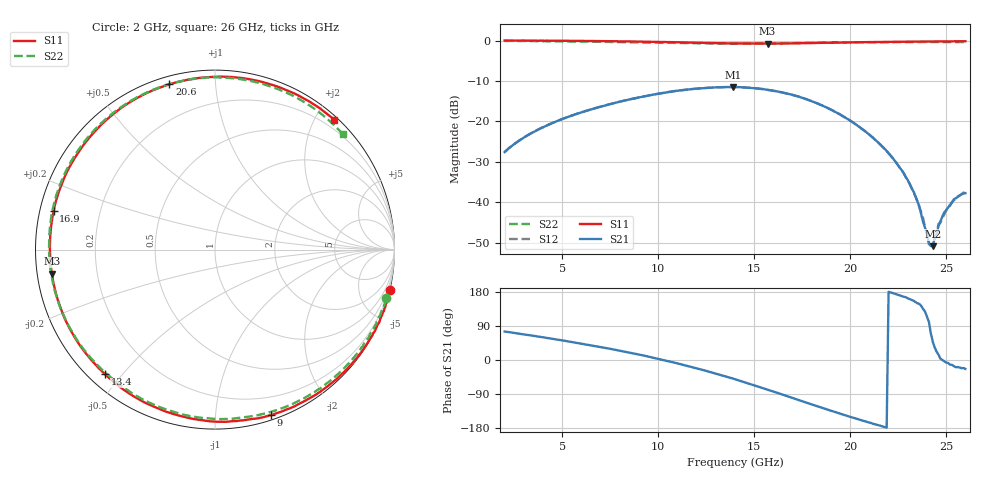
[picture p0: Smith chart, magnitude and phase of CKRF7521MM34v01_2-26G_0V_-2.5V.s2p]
! CHUO DENSHI KOGYO Co.,Ltd.
! 1. March 2016
! CKRF7521MM34
! N-channel HJ-FET
! Vds = 0 V Vgs = -2.5 V
# Hz S  MA  R 50
!  f  S11  S21  S12  S22
!  Hz  MAG  ANG  MAG  ANG  MAG  ANG  MAG  ANG
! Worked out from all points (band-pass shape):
!   241 points, 2 GHz to 26 GHz, reference 50 ohm
!   highest |S21| = -11.48 dB at 13.9 GHz (marker M1); lowest = -50.9 dB at 24.3 GHz (marker M2)
!   |S21| within 3 dB of the highest: 8.573 GHz to 17.71 GHz (9.138 GHz wide, 69.5 % of centre)
!   lowest |S11| = -0.7 dB at 15.7 GHz (marker M3), VSWR 23.56, Z = 2.13 - j3.69 ohm
!   |S11| at or under -10 dB: nowhere
!   |S22| runs from -0.7 to -0.1 dB; largest |S21 - S12| = 0.00066
!   S11 on the Smith chart (normalised r, x): 2 GHz: -0.06, -8.68; 9 GHz: 0.04, -1.39; 13.4 GHz: 0.05, -0.45; 16.9 GHz: 0.04, +0.12; 20.6 GHz: 0.04, +0.76; 26 GHz: 0.05, +2.28
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2e9  1.002 -13.1  0.04171 75.2  0.04194 75.2  0.9908 -15.9
3.8e9  0.999 -25.6  0.08043 61.5  0.08046 61.5  0.9834 -30.5
6e9  0.9913 -42.7  0.1294 43.3  0.1297 43.3  0.9724 -49.4
9e9  0.9729 -71.4  0.1985 14.4  0.1985 14.4  0.9497 -78.5
1e10  0.963 -82.9  0.2202 3.3  0.22 3.2  0.9433 -89.3
1.18e10  0.9432 -106.8  0.252 -19.3  0.2521 -19.3  0.929 -110.8
1.34e10  0.9262 -131.4  0.2655 -41.6  0.2658 -41.7  0.9181 -132.0
1.39e10  0.9228 -139.7  0.2667 -49.3  0.2667 -49.3  0.9186 -139.1
1.4e10  0.9231 -141.3  0.2661 -50.9  0.2662 -50.9  0.9181 -140.5
1.57e10  0.9186 -171.5  0.2461 -78.3  0.246 -78.2  0.9213 -166.5
1.69e10  0.9246 166.6  0.2162 -98.4  0.216 -98.3  0.9267 173.9
1.8e10  0.9334 146.9  0.1779 -117.3  0.1779 -117.2  0.9368 155.5
1.93e10  0.9455 125.0  0.1282 -138.7  0.1281 -138.8  0.9467 133.7
2.06e10  0.9553 105.4  0.08142 -159.2  0.08122 -159.0  0.9541 112.7
2.2e10  0.9647 86.9  0.04041 179.9  0.0403 -179.8  0.9596 91.6
2.33e10  0.971 72.2  0.01352 156.4  0.01338 156.6  0.9608 73.7
2.38e10  0.9731 67.0  0.005678 134.6  0.006334 134.4  0.9604 67.4
2.41e10  0.9749 64.1  0.003132 100.4  0.003023 96.5  0.9608 63.6
2.43e10  0.9761 62.2  0.002856 48.5  0.003042 53.9  0.9608 61.2
2.46e10  0.9767 59.4  0.005061 14.0  0.005403 15.6  0.9602 57.7
2.49e10  0.9784 56.7  0.007509 -3.7  0.007039 -2.3  0.9606 54.1
2.6e10  0.9831 47.4  0.01292 -23.5  0.01303 -22.3  0.9599 42.1
